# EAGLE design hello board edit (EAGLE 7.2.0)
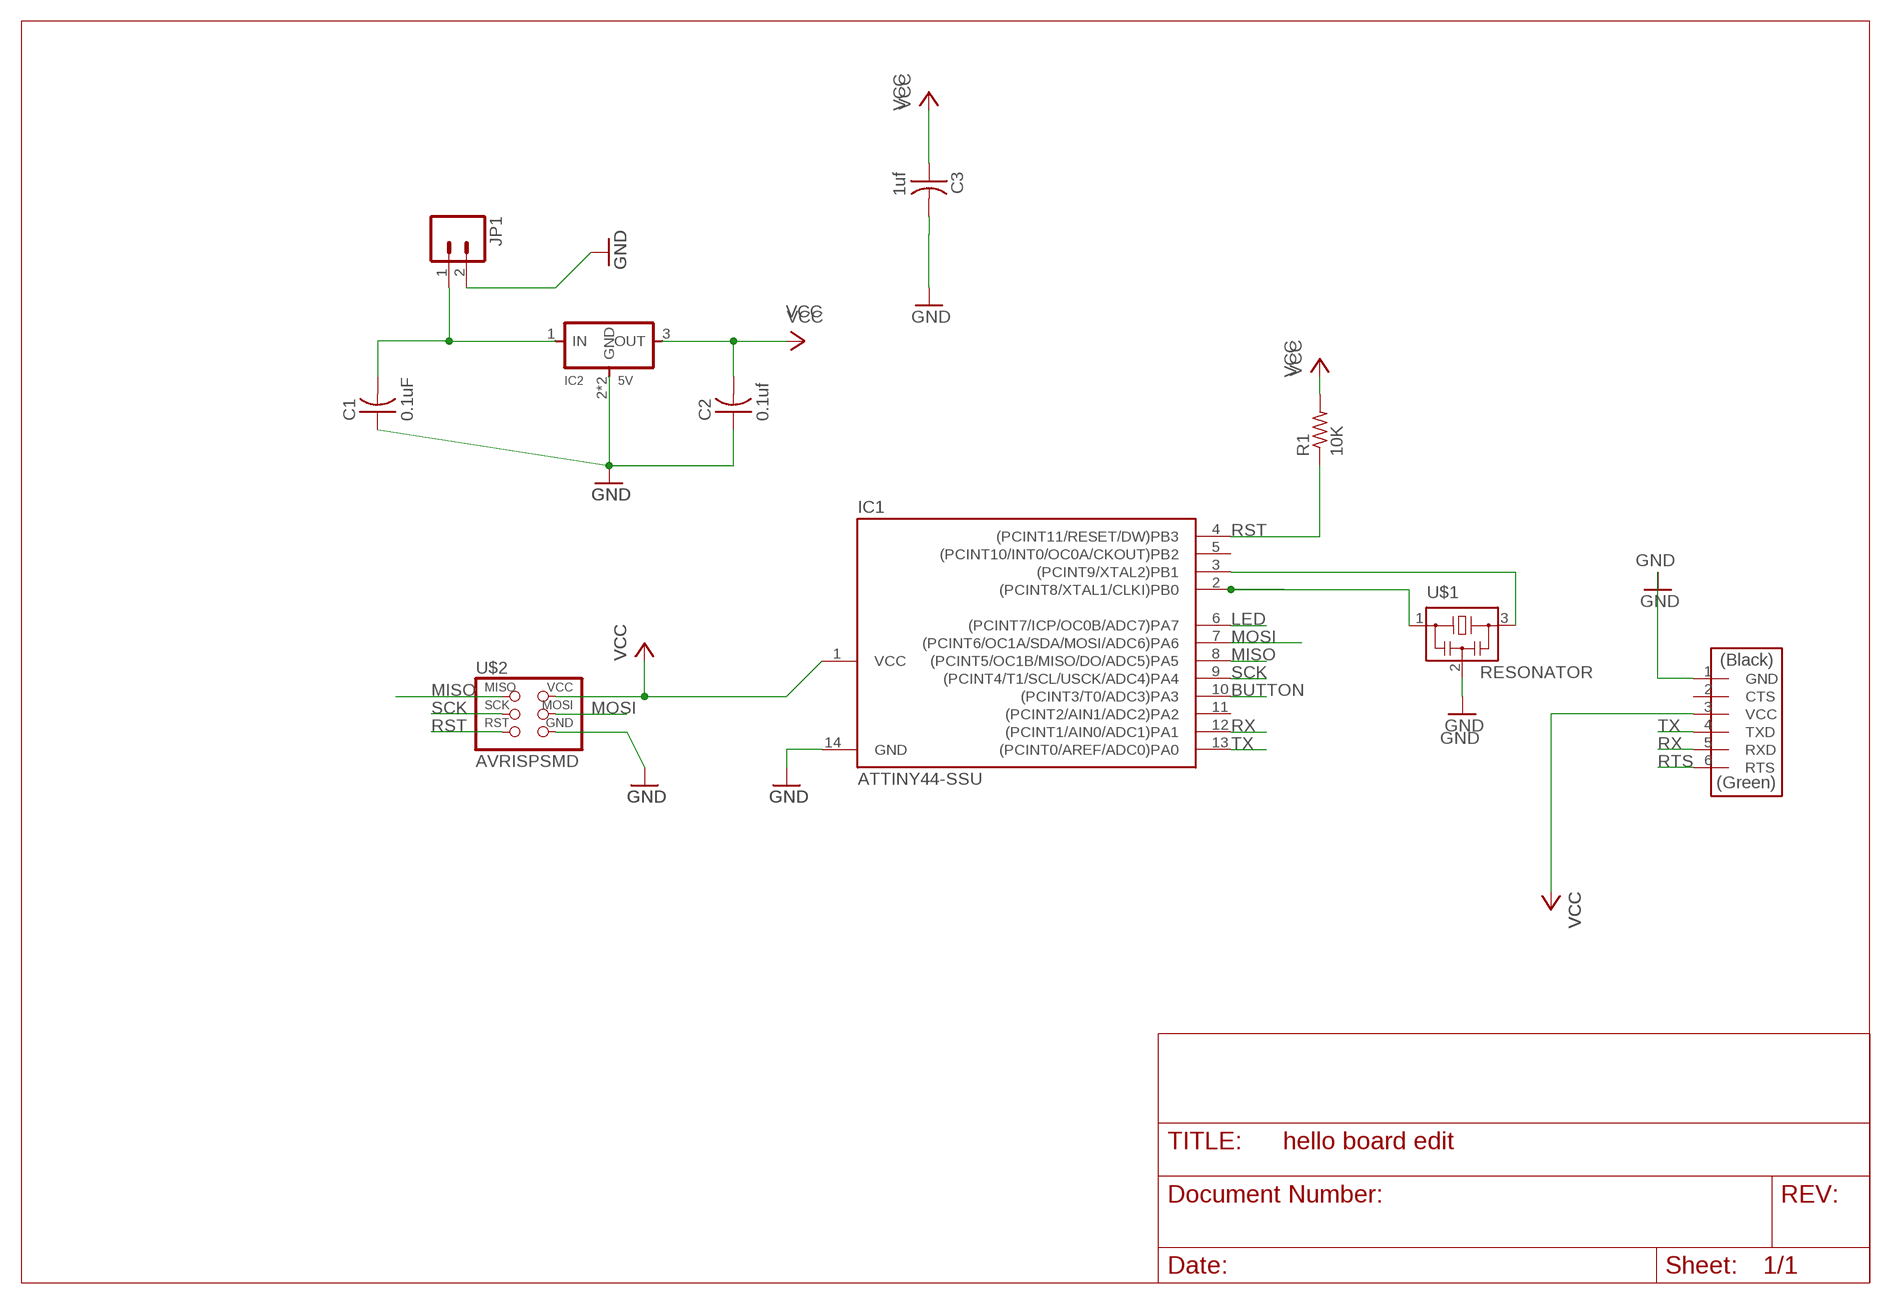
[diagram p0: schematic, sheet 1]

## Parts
C1  0.1uF  CAP-US1206FAB  [C1206FAB]
C2  0.1uf  CAP-US1206FAB  [C1206FAB]
C3  1uf  CAP-US1206FAB  [C1206FAB]
IC1  ATTINY44-SSU  [SOIC14]
IC2  5V  REGULATORSOT223  [SOT223]
JP1  M02LOCK  [1X02_LOCK]
R1  10K  RES-US1206FAB  [R1206FAB]
U$1  RESONATOR  [EFOBM]
U$2  AVRISPSMD  [2X03SMD]
U$3  FTDI-SMD-HEADER  [1X06SMD]

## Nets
BUTTON: IC1.10((PCINT3/T0/ADC3)PA3)
GND: C1.1 C2.1 C3.2 IC1.14(GND) IC2.2(GND) IC2.4(GND) JP1.2 U$1.2 U$2.6(GND) U$3.1(GND)
LED: IC1.6((PCINT7/ICP/OC0B/ADC7)PA7)
MISO: IC1.8((PCINT5/OC1B/MISO/DO/ADC5)PA5) U$2.1(MISO)
MOSI: IC1.7((PCINT6/OC1A/SDA/MOSI/ADC6)PA6) U$2.4(MOSI)
N$1: IC1.3((PCINT9/XTAL2)PB1) U$1.3
N$3: IC1.2((PCINT8/XTAL1/CLKI)PB0) U$1.1
N$4: C1.2 IC2.1(IN) JP1.1
RST: IC1.4((PCINT11/RESET/DW)PB3) R1.1 U$2.5(RST)
RTS: U$3.6(RTS)
RX: IC1.12((PCINT1/AIN0/ADC1)PA1) U$3.5(RXD)
SCK: IC1.9((PCINT4/T1/SCL/USCK/ADC4)PA4) U$2.3(SCK)
TX: IC1.13((PCINT0/AREF/ADC0)PA0) U$3.4(TXD)
VCC: C2.2 C3.1 IC1.1(VCC) IC2.3(OUT) R1.2 U$2.2(VCC) U$3.3(VCC)
Unconnected: IC1.5((PCINT10/INT0/OC0A/CKOUT)PB2) IC1.11((PCINT2/AIN1/ADC2)PA2) U$3.2(CTS)

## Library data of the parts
C1-C3 = 01_fab:CAP-US
IC1 = 01_fab:ATTINY44
IC2 = 01_fab:REGULATOR
JP1 = 01_SparkFun:M02: Header 2
R1 = 01_fab:RES-US: Resistor (US Symbol)
U$1 = 01_fab:RESONATOR
U$2 = 01_fab:AVRISP
U$3 = 01_fab:FTDI-SMD-HEADER

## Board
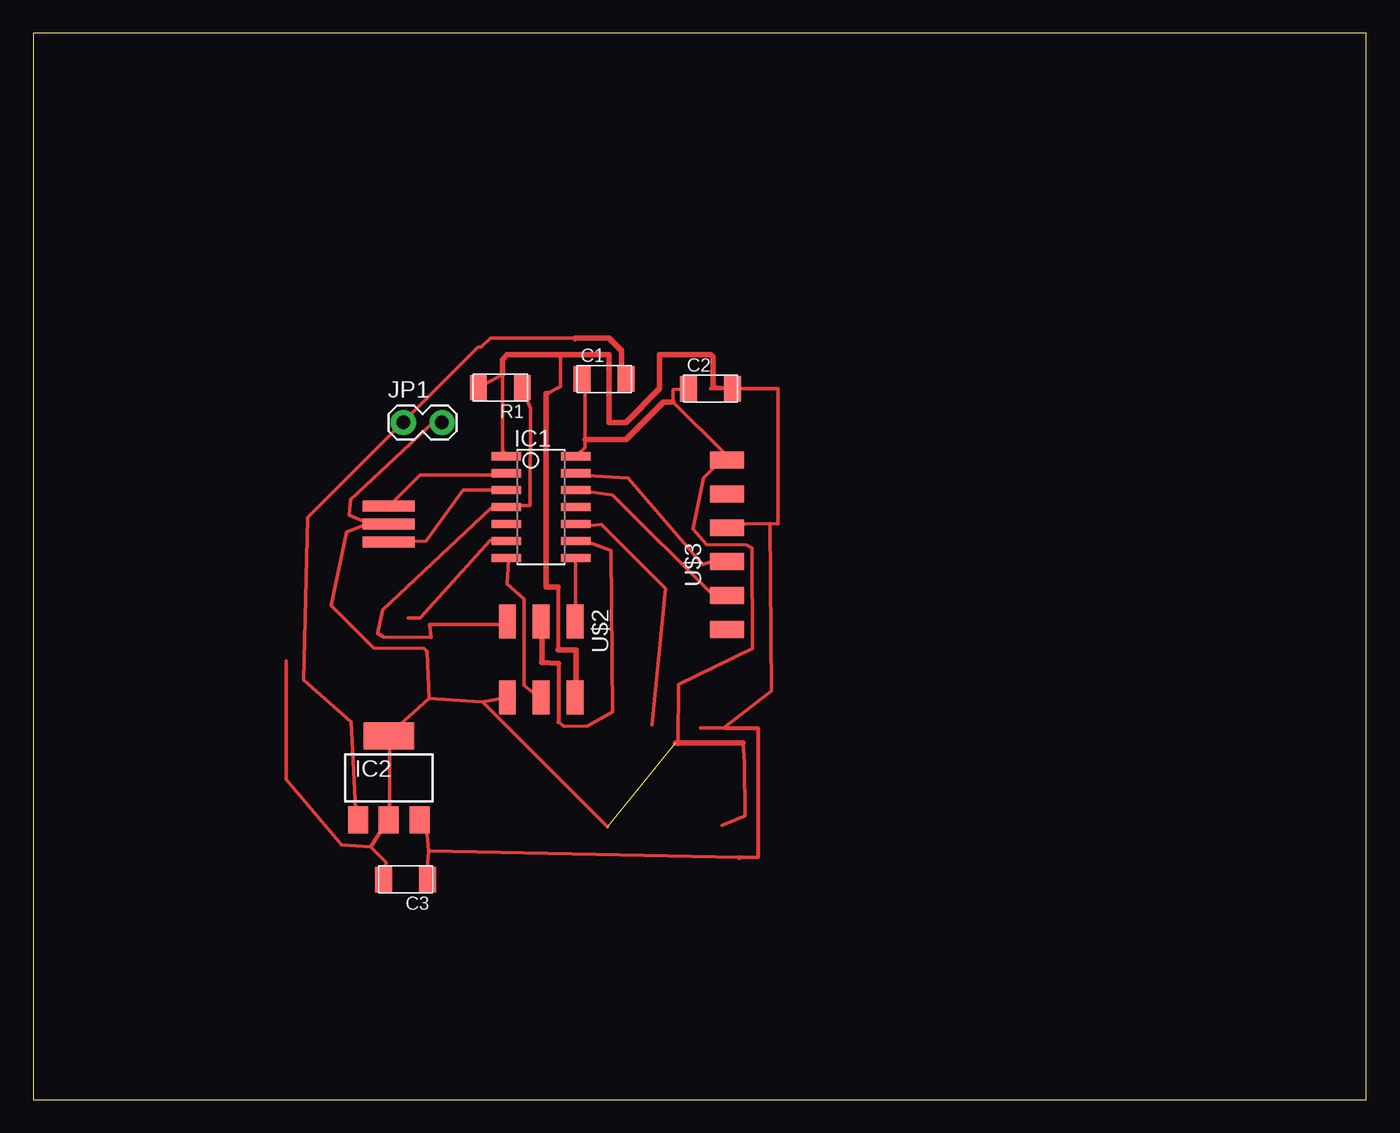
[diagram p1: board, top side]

Size 100 x 80 mm. Coordinates in mm from the lower left corner, seen from the top.
Outline: 0,0 100,0 100,80 0,80 0,0
Copper layers (1*16): Top 0.035mm / dielectric 1.5mm / Bottom 0.035mm
Design rules "fabmodule": minimum track width 10mil, minimum drill 0.4mm, track to track 0.42mm, track to pad 0.42mm, pad to pad 0.42mm, via to via 0.42mm, smd to smd 0.42mm, copper to edge 40mil, drill to drill 0.8mm, minimum pad ring 10mil, minimum via ring 8mil, stop-mask expansion 4mil, vias tented up to drill 0mil, thermal gap 10mil

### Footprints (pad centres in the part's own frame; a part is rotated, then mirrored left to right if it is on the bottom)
C1206FAB = smd 1.27 x 1.905: 1 -1.651,0; 2 1.651,0
SOIC14 = smd 0.61 x 2.21: 1 -3.81,-2.603; 2 -2.54,-2.603; 3 -1.27,-2.603; 4 0,-2.603; 5 1.27,-2.603; 6 2.54,-2.603; 7 3.81,-2.603; 8 3.81,2.603; 9 2.54,2.603; 10 1.27,2.603; 11 0,2.603; 12 -1.27,2.603; 13 -2.54,2.603; 14 -3.81,2.603
SOT223 = smd 1.5 x 2: 1 -2.3,-3.15; 2 0,-3.15; 3 2.3,-3.15 | smd 3.8 x 2: 4 0,3.15
1X02_LOCK = drill 1.016 pad 1.88: 1 -0.178,0; 2 2.718,0
R1206FAB = smd 1.27 x 1.905: 1 -1.651,0; 2 1.651,0
EFOBM = smd 0.8 x 3.9: 1 -1.35,0; 2 0,0; 3 1.35,0
2X03SMD = smd 2.54 x 1.27: 1 -2.857,2.54; 2 2.857,2.54; 3 -2.857,0; 4 2.857,0; 5 -2.857,-2.54; 6 2.857,-2.54
1X06SMD = smd 2.54 x 1.27: 1 0,6.35; 2 0,3.81; 3 0,1.27; 4 0,-1.27; 5 0,-3.81; 6 0,-6.35

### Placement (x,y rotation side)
C1  42.83,54.07 0 top
C2  50.8,53.34 0 top
C3  27.94,16.51 180 top
IC1  38.1,44.45 270 top
IC2  26.67,24.13 0 top
JP1  27.94,50.8 0 top
R1  35.04,53.42 180 top
U$1  26.67,43.18 270 top
U$2  38.1,33.02 270 top
U$3  52.05,41.63 0 top

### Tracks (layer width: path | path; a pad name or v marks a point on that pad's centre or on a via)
BUTTON
  Top 0.254: 46.41,28.12 47.45,38.34 42.65,43.14 40.92,42.98 IC1.10
GND  (1 unrouted)
  Top 0.254: 18.97,32.92 18.97,24 23.15,19.12 25.31,18.95 | 25.31,18.95 26.52,20.8 IC2.2 26.75,21.03 26.75,27.2 IC2.4 26.75,27.43 29.7,30.09 | C3.2 26.45,17.81 25.31,18.95 | C1.1 41.38,53.26 41.38,49.53 41.38,48.92 40.92,48.46 IC1.14 | C2.1 48.01,53.26 48.01,52.35 51.89,48.46 U$3.1 51.89,48.23 50.29,46.63 49.48,42.82 50.5,41.64 53.49,41.6 53.9,41.38 53.95,33.84 48.41,31.15 48.38,26.73 | 25.15,43.2 23.7,43.87 23.81,45.03 29.95,50.75 30.63,50.75 JP1.2 | 25.15,43.2 26.52,43.2 U$1.2 25.15,43.2 | 29.7,30.09 33.71,29.83 | 33.71,29.83 43.08,20.46 | 33.71,29.83 U$2.6 | 25.15,43.2 23.52,42.57 22.33,37.08 25.54,33.88 29.31,33.85 29.54,33.62 29.7,30.09 | 53.23,26.76 53.36,25.3 53.4,21.28 51.66,20.57
  Top 0.406: 48.01,52.35 47.27,52.35 44.45,49.53 41.38,49.53 | 53.23,26.76 48.18,26.76 48.38,26.73
LED
  Top 0.254: 28.12,36.12 29.03,36.12 34.28,41.95 35.43,41.83 IC1.6
MISO
  Top 0.254: IC1.8 40.69,40.46 40.69,35.89 U$2.1
MOSI
  Top 0.254: IC1.7 35.66,40.46 35.55,38.69 36.8,37.56 36.8,31.07 37.95,30.18 U$2.4
N$1
  Top 0.254: IC1.3 32.23,45.72 29.48,41.9 26.75,41.83 U$1.3
N$3
  Top 0.254: IC1.2 35.43,46.86 29.03,46.86 26.75,44.58 U$1.1
N$4
  Top 0.254: 44.12,53.49 44.81,53.49 C1.2 | IC2.1 24.23,21.03 23.84,28.33 20.29,31.49 20.57,43.66 27.66,50.75 JP1.1 27.89,50.98 33.38,56.46 33.6,56.46 34.29,57.15 40.64,57.15 40.64,56.97
  Top 0.406: 44.12,53.49 44.12,56.21 43.18,57.15 40.64,57.15
RST
  Top 0.254: R1.1 37.31,51.83 37.27,44.58 36.35,44.58 35.66,44.58 IC1.4 35.43,44.35 34.29,44.35 26.2,36.74 25.85,34.98 26.29,34.7 29.83,34.66 29.72,35.66 35.43,35.66 U$2.5
RX
  Top 0.254: IC1.12 43.47,45.36 51.02,37.81 U$3.5
SCK
  Top 0.254: 39.39,28.32 39.82,27.98 41.58,28.02 43.45,29.1 43.36,41.2 41.6,41.83 40.92,41.83 IC1.9 | 38.18,35.2 38.18,35.66 U$2.3
  Top 0.305: 39.39,32.72 39.39,28.32
  Top 0.406: 39.39,32.72 38.12,32.77 38.12,32.8 38.18,32.8 38.18,35.2
TX
  Top 0.254: IC1.13 40.92,46.86 44.62,46.63 50.21,40.13 51.89,40.69 U$3.4
VCC
  Top 0.254: R1.2 35.2,54.41 35.2,48.69 35.43,48.46 IC1.1 | 38.54,52.97 39.55,53.49 39.55,55.78 | 40.46,30.18 U$2.2 | 29.65,18.67 29.49,20.34 29.03,20.8 IC2.3 | 29.65,18.67 29.49,16.69 C3.1 | 52.97,18.17 29.65,18.67 | 50.06,27.89 51.89,27.89 51.9,27.97 55.37,30.64 55.29,43.2 | 50.98,53.49 C2.2 | C2.2 50.8,53.34 | C2.2 55.88,53.34 55.88,43.18 55.29,43.2 | 55.29,43.2 53.34,43.18 53.25,43.14 52.23,43.14 U$3.3
  Top 0.305: 39.35,38.46 39.35,33.73 | 51.89,27.89 arc90 51.91,27.87 54.36,27.87 | 54.36,27.87 54.36,18.19 52.97,18.12 52.97,18.17 | 54.36,27.87
  Top 0.406: 35.2,54.41 35.2,55.52 35.56,55.88 39.45,55.88 39.55,55.78 39.65,55.88 43.18,55.88 43.18,50.8 44.45,50.8 46.99,53.34 46.99,55.88 50.8,55.88 50.98,55.7 50.98,53.49 | 40.46,30.18 40.72,30.18 40.72,33.73 39.35,33.73 | 38.54,52.97 38.46,52.97 38.46,38.46 39.35,38.46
